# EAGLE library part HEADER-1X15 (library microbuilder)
1x15 Header
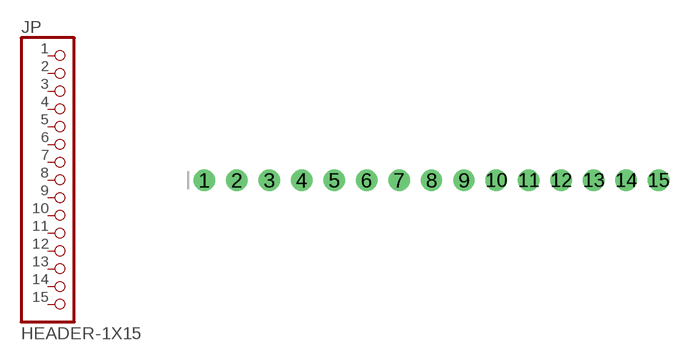
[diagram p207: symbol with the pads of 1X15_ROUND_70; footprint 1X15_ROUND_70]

Designator prefix JP

## HEADER-1X15  [1X15_ROUND_70]
1  1  pas
2  2  pas
3  3  pas
4  4  pas
5  5  pas
6  6  pas
7  7  pas
8  8  pas
9  9  pas
10  10  pas
11  11  pas
12  12  pas
13  13  pas
14  14  pas
15  15  pas

## Footprint 1X15_ROUND_70 (pad centres in mm)
drill 1 pad 1.676: 1 -17.78,0; 2 -15.24,0; 3 -12.7,0; 4 -10.16,0; 5 -7.62,0; 6 -5.08,0; 7 -2.54,0; 8 0,0; 9 2.54,0; 10 5.08,0; 11 7.62,0; 12 10.16,0; 13 12.7,0; 14 15.24,0; 15 17.78,0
